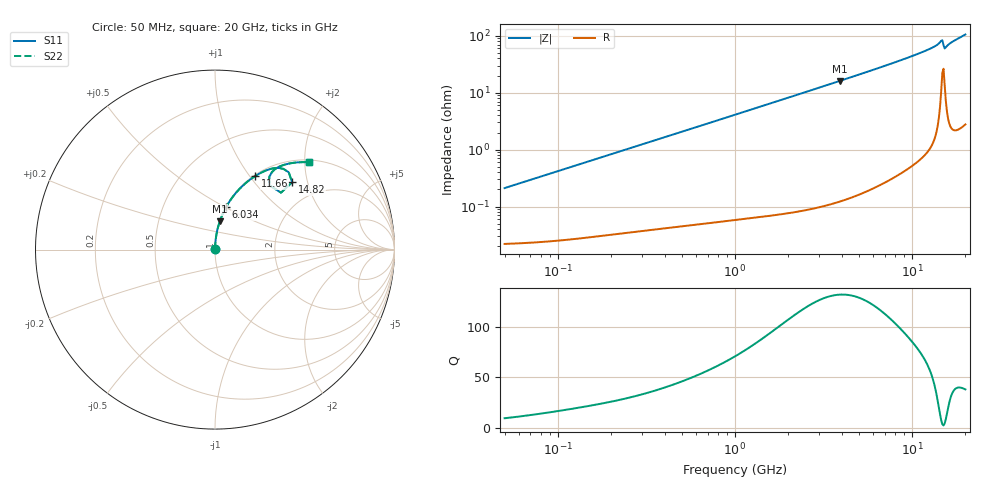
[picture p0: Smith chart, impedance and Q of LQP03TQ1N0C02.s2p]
!Murata Part Number: LQP03TQ1N0C02
!These Parameters are Measured in Series Mode Connection
!  o--[Z]--o
!Port1  Port2
!  o-------o
!Freq. Start=50[MHz] Stop=20[GHz], 401[Steps]
# Hz S RI R 50
!Freq.(Hz) S11(Real) S11(Imag) S21(Real) S21(Imag) S12(Real) S12(Imag) S22(Real) S22(Imag)
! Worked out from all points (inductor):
!   401 points, 50 MHz to 20 GHz, reference 50 ohm
!   read as one part in series: L = 668 pH near 51.52 MHz
!   highest Q = 132 at 3.908 GHz (marker M1), where L = 656 pH
!   S11 on the Smith chart (normalised r, x): 50 MHz: 1.00, +0.00; 6.034 GHz: 1.00, +0.51; 11.66 GHz: 1.02, +1.06; 14.82 GHz: 1.45, +1.61; 20 GHz: 1.06, +2.11
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5e7  0.000225 0.0021  0.9998 -0.0021  0.9998 -0.0021  0.000225 0.0021
1.364002e8  0.00031 0.00569  0.9997 -0.00569  0.9997 -0.00569  0.00031 0.00569
3.721004e8  0.000638 0.0153  0.9994 -0.0153  0.9994 -0.0153  0.000638 0.0153
1e9  0.00225 0.0409  0.9977 -0.0409  0.9977 -0.0409  0.00225 0.0409
1.714689e9  0.00561 0.0698  0.9944 -0.0698  0.9944 -0.0698  0.00561 0.0698
2.728004e9  0.0133 0.1104  0.9867 -0.1104  0.9867 -0.1104  0.0133 0.1104
3.908127e9  0.0265 0.1567  0.9735 -0.1567  0.9735 -0.1567  0.0265 0.1567
6.034176e9  0.0617 0.2366  0.9383 -0.2366  0.9383 -0.2366  0.0617 0.2366
7.442007e9  0.093 0.2858  0.907 -0.2858  0.907 -0.2858  0.093 0.2858
9.457416e9  0.1483 0.3498  0.8517 -0.3498  0.8517 -0.3498  0.1483 0.3498
1.166392e10  0.2237 0.4095  0.7763 -0.4095  0.7763 -0.4095  0.2237 0.4095
1.295331e10  0.2784 0.4385  0.7216 -0.4385  0.7216 -0.4385  0.2784 0.4385
1.396067e10  0.3386 0.4548  0.6614 -0.4548  0.6614 -0.4548  0.3386 0.4548
1.438523e10  0.381 0.4498  0.619 -0.4498  0.619 -0.4498  0.381 0.4498
1.460232e10  0.411 0.4305  0.589 -0.4305  0.589 -0.4305  0.411 0.4305
1.482269e10  0.4297 0.3752  0.5703 -0.3752  0.5703 -0.3752  0.4297 0.3752
1.527346e10  0.3041 0.358  0.6959 -0.358  0.6959 -0.358  0.3041 0.358
1.550395e10  0.3024 0.4049  0.6976 -0.4049  0.6976 -0.4049  0.3024 0.4049
1.573793e10  0.3168 0.4314  0.6832 -0.4314  0.6832 -0.4314  0.3168 0.4314
1.621653e10  0.3479 0.4568  0.6521 -0.4568  0.6521 -0.4568  0.3479 0.4568
1.696185e10  0.3887 0.4735  0.6113 -0.4735  0.6113 -0.4735  0.3887 0.4735
2e10  0.5262 0.4863  0.4738 -0.4863  0.4738 -0.4863  0.5262 0.4863
